PROGRAM MAIN
VAR
	// control of the program
	bStart : BOOL;
	Mode	: E_WriteMode; 
	nState : INT; 
	bError : BOOL := FALSE;
	sError: T_MAXSTRING;

	// fb to control the data communication
	fbCSV_Access: FB_CSV_Access;
	InputData : ST_CSVDataStruct;
	
	// datageneration
	rand: DRAND;
	randomNumber: LREAL;
	fbGetSystemTime: GETSYSTEMTIME;
	fileTime : T_FILETIME;
	
	// repetition
	Count: INT;
	ValuesToWrite: INT := 1000;
	risingTrigger: R_TRIG;
	
	// measure time to execute actions
	Timer : TON;
	t : TIME; 
	
	// destination array of read data
	ReadData: ARRAY[0..4] OF ST_CSVDataStruct;
		
	
END_VAR

Timer(); 

CASE nState OF 
	
	
	0: // init
 
		Count := 0;
		GenerateData();
		Timer (IN:= FALSE);
		risingTrigger(CLK:= bStart);
		
		IF risingTrigger.Q THEN
			
			bStart := FALSE;
			bError := FALSE;
			sError := '';
			
			Timer (IN:= TRUE, PT := T#1H);
			
			IF mode = E_WriteMode.ePLCDBCmd THEN
				nState := 1;
				
			ELSIF mode = E_WriteMode.ePLCDBWriteStruct THEN
				nState := 11;
				
			ELSIF mode = E_WriteMode.ePLCDBReadStruct THEN
				nState := 21;
				
			END_IF
						
		END_IF
		
	
	1:  // fb_PLCDBCMD
	
		IF fbCSV_Access.Write(3, InputData) THEN
			
			IF fbCSV_Access.bError THEN
				nState := 255;
			ELSE
				Count:= Count+1;
				nState := 2; 
			END_IF	
		
		END_IF

		
	2: // repetitions
		
		IF Count <= ValuesToWrite THEN
			GenerateData(); 
			nState := 1;
		ELSE
			t := Timer.ET;
			nState := 0;
		END_IF
	
	
	11: // fbPLCDBWriteStruct
	
		IF fbCSV_Access.WriteStruct(1, InputData) THEN
			IF fbCSV_Access.bError THEN
				nState := 255;
			ELSE
				Count:= Count+1;
				nState := 12; 
			END_IF		
		END_IF		
		
		
	12: // repetitions
	
		IF Count <= ValuesToWrite THEN
			GenerateData(); 
			nState := 11;
		ELSE
			t := Timer.ET;
			nState := 0;
		END_IF

   
	21:  // fbPLCDBReadStruct
	
		IF fbCSV_Access.ReadStruct(hDBID := 1, pData := ADR(ReadData), cbData := SIZEOF(ReadData)) THEN
			IF fbCSV_Access.bError THEN
				nState := 255;
			ELSE
				nState := 0; 
			END_IF		
		END_IF

	
	255: // error
	
		// request error text
		fbCSV_Access.ipTcResult.RequestEventText(1033, sError, SIZEOF(sError));
		bError := TRUE;

END_CASE

METHOD GenerateData : BOOL
VAR_INPUT
END_VAR

VAR
	
END_VAR
rand(Seed := 1, Num => randomNumber);

InputData.ID := InputData.ID +1; 

InputData.Temperature :=InputData.Temperature  + ((randomNumber-0.5)*10)/5;

rand(Seed := 1, Num => randomNumber);
InputData.Velocity := InputData.Velocity + (randomNumber-0.5);

fbGetSystemTime(timeLoDW => fileTime.dwLowDateTime, timeHiDW => fileTime.dwHighDateTime);
InputData.Timestamp := FILETIME_TO_DT(fileTime);

InputData.Name := 'Water Turbine';
END_METHOD

END_PROGRAM
